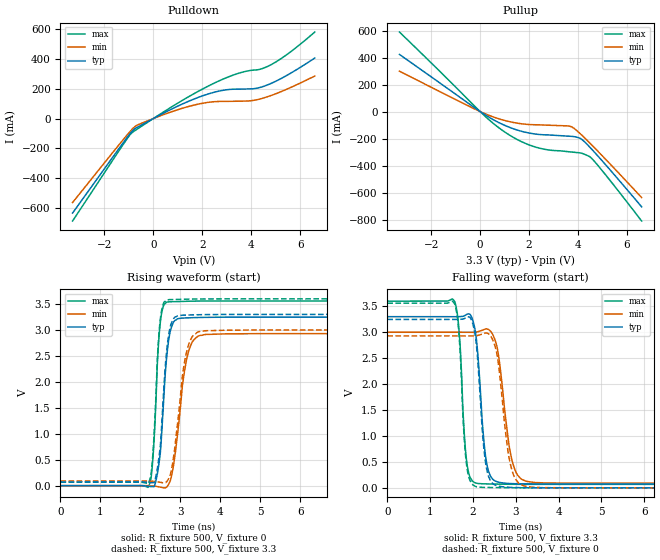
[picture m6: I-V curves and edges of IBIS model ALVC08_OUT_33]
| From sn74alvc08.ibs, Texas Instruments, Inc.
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[Model]   ALVC08_OUT_33
Model_type  Output
Vref =   0
Rref =   500
Cref =   50p
Vmeas =   1.5
| variable   typ   min   max
C_comp   7.53pF   5.16pF   11.40pF
| C_pullup   8.40pF   6.43pF   11.40pF
| C_pulldown   6.66pF   5.16pF   9.51pF
[Temperature Range]   40   100   -40
| Ambient temperature   25   85   -40
[Voltage range]   3.3   3   3.6
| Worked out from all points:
|   slope of the pulldown table from 0 to 0.495 V, typ, clamps not added: 11.6 ohm
|   slope of the pullup table from 0 to 0.495 V, typ, clamps not added: 8.84 ohm
|   rising waveform, R_fixture 500, V_fixture 0: 20-80 % time 174ps typ, 269ps min, 135ps max; typ from 0 V to 3.25 V
|   falling waveform, R_fixture 500, V_fixture 3.3: 20-80 % time 174ps typ, 255ps min, 133ps max; typ from 3.3 V to 0.073 V
|   rising waveform, R_fixture 500, V_fixture 3.3: 20-80 % time 174ps typ, 263ps min, 135ps max; typ from 0.073 V to 3.3 V
|   falling waveform, R_fixture 500, V_fixture 0: 20-80 % time 171ps typ, 241ps min, 135ps max; typ from 3.25 V to 0 V
[Pulldown]
| ALVC08_OUT_33
|   Voltage   I(typ)   I(min)   I(max)
-3.3V     -631.7mA   -561.5mA   -685mA
-1.115V   -136.4mA   -118.3mA   -145.6mA
-910mV    -93.12mA   -79.48mA   -100.6mA
-740mV    -66.58mA   -52.27mA   -79.35mA
825mV     69.55mA    49.91mA    85.75mA
2.12V     157.8mA    105.3mA    206.7mA
2.98V     192.3mA    114.9mA    272.7mA
3.985V    198.5mA    119.1mA    321.9mA
4.4V      209.9mA    132.7mA    331.5mA
4.855V    238mA      156.6mA    363.9mA
5.605V    302.5mA    207mA      445.3mA
6.6V      404.7mA    284.5mA    578.6mA
[Pullup]
| ALVC08_OUT_33
|   Voltage   I(typ)   I(min)   I(max)
-3.3V     423.4mA    299.2mA    589.2mA
100mV     -12.23mA   -8.248mA   -17.57mA
950mV     -97.85mA   -63.56mA   -144.6mA
1.595V    -141.3mA   -88.12mA   -214.5mA
2.245V    -166.3mA   -97.73mA   -262.1mA
2.8V      -173.2mA   -101.1mA   -284.5mA
3.75V     -183.9mA   -114.4mA   -299.9mA
4.115V    -201.1mA   -168.2mA   -307.3mA
4.435V    -254.9mA   -224.6mA   -330.1mA
4.555V    -278.1mA   -246.5mA   -346.3mA
5.24V     -417.4mA   -374.9mA   -494.4mA
6.6V      -705.7mA   -637.2mA   -810.8mA
[Ramp]
| ALVC08_OUT_33
| variable   typ   min   max
dV/dt_r   1.96/1.77E-10   1.78/2.87E-10   2.16/1.42E-10
dV/dt_f   1.97/1.84E-10   1.79/2.76E-10   2.15/1.41E-10
R_load = 500
[Rising Waveform]
| ALVC08_OUT_33
R_fixture =   500
C_fixture =   0
L_fixture =   0
V_fixture =   0
V_fixture_min = 0
V_fixture_max = 0
|   Time   V(typ)   V(min)   V(max)
0s        40.4pV     4.177nV    33.01pV
2.2ns     -13.29mV   -555.7uV   -26mV
2.315ns   -18.73mV   -5.324mV   533.1mV
2.43ns    248.1mV    -17.14mV   2.41V
2.505ns   676.9mV    -27.97mV   3.179V
2.63ns    2.213V     -40.87mV   3.517V
2.73ns    2.9V       60.97mV    3.545V
3.185ns   3.234V     2.521V     3.554V
3.64ns    3.244V     2.914V     3.559V
50ns      3.247V     2.929V     3.56V
[Falling Waveform]
| ALVC08_OUT_33
R_fixture =   500
C_fixture =   0
L_fixture =   0
V_fixture =   3.3
V_fixture_min = 3
V_fixture_max = 3.6
|   Time   V(typ)   V(min)   V(max)
0s        3.3V       3V         3.6V
1.575ns   3.299V     3V         3.589V
1.685ns   3.301V     3V         2.92V
1.855ns   3.346V     2.999V     491.7mV
2.14ns    2.276V     3.016V     81.28mV
2.27ns    771.9mV    3.056V     76.33mV
2.405ns   231.8mV    3.026V     73.78mV
2.93ns    80.05mV    469.3mV    67.74mV
3.425ns   73.29mV    102.8mV    66.32mV
50ns      72.86mV    89.69mV    66.1mV
[Rising Waveform]
| ALVC08_OUT_33
R_fixture =   500
C_fixture =   0
L_fixture =   0
V_fixture =   3.3
V_fixture_min = 3
V_fixture_max = 3.6
|   Time   V(typ)   V(min)   V(max)
0s        72.86mV    89.69mV    66.1mV
2.195ns   60.62mV    89.18mV    35.7mV
2.31ns    58.22mV    84.99mV    567.6mV
2.43ns    350.6mV    74.43mV    2.497V
2.5ns     762.2mV    65.95mV    3.208V
2.625ns   2.303V     57.57mV    3.556V
2.725ns   2.972V     163.2mV    3.586V
3.17ns    3.288V     2.615V     3.594V
3.63ns    3.297V     2.986V     3.599V
50ns      3.3V       3V         3.6V
[Falling Waveform]
| ALVC08_OUT_33
R_fixture =   500
C_fixture =   0
L_fixture =   0
V_fixture =   0
V_fixture_min = 0
V_fixture_max = 0
|   Time   V(typ)   V(min)   V(max)
0s        3.247V     2.929V     3.56V
1.575ns   3.247V     2.929V     3.543V
1.675ns   3.248V     2.929V     2.936V
1.855ns   3.291V     2.929V     410.9mV
2.045ns   2.978V     2.929V     31.68mV
2.155ns   1.923V     2.948V     11.47mV
2.405ns   141.5mV    2.937V     5.722mV
2.89ns    7.709mV    398.3mV    1.764mV
3.375ns   657.9uV    11.57mV    253.5uV
50ns      41.42pV    4.178nV    33.76pV
